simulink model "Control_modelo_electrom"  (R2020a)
settings: Solver=VariableStepAuto  StartTime=0.0  StopTime=10.0  RelTol=1e-3
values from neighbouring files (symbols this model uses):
  b = 0.1    [Comando_linmod.m]
  k = 0.8    [Comando_linmod.m]
  kf = 0.45    [Comando_linmod.m]
  kv = 0.45    [Comando_linmod.m]
  L = 0.1    [Comando_linmod.m]
  m = 0.15    [Comando_linmod.m]
  M = 5    [Comando_linmod.m]
  R = 0.25    [Comando_linmod.m]
undefined symbols (not defined in the file or in its folder): den, num
libraries: simulink x2

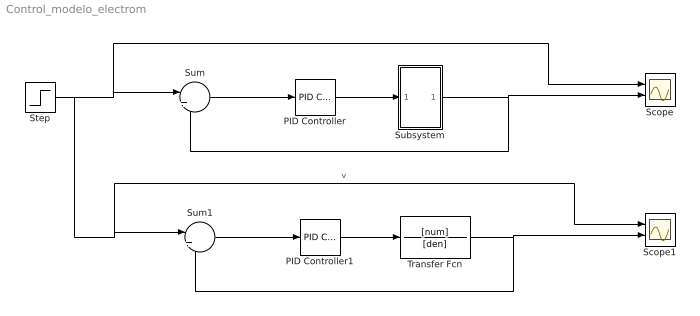
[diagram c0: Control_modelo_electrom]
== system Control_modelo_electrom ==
  PID Controller : simulink/Continuous/PID Controller  Controller=PID  Form=Parallel  TimeDomain=Continuous-time  UseExternalTs=off  SampleTime=-1  IntegratorMethod=Forward Euler  FilterMethod=Forward Euler  ControllerParametersSource=internal  P=1  I=1  D=0  UseFilter=on  N=100  TunerSelectOption=Transfer Function Based (PID Tuner App)  InitialConditionSource=internal  InitialConditionForIntegrator=0  InitialConditionForFilter=0  DifferentiatorICPrevScaledInput=0  ExternalReset=none  TrackingMode=off  Kt=1  LimitOutput=off  UpperSaturationLimit=inf  LowerSaturationLimit=-inf  LinearizeAsGain=on  AntiWindupMode=none  Kb=1  POutMin=[]  POutMax=[]  IOutMin=[]  IOutMax=[]  DOutMin=[]  DOutMax=[]  NOutMin=[]  NOutMax=[]  SumOutMin=[]  SumOutMax=[]  SaturationOutMin=[]  SaturationOutMax=[]  PParamMin=[]  PParamMax=[]  IParamMin=[]  IParamMax=[]  DParamMin=[]  DParamMax=[]  NParamMin=[]  NParamMax=[]  KbParamMin=[]  KbParamMax=[]  KtParamMin=[]  KtParamMax=[]  KbOutMin=[]  KbOutMax=[]  KtOutMin=[]  KtOutMax=[]  IntegratorOutMin=[]  IntegratorOutMax=[]  FilterOutMin=[]  FilterOutMax=[]  SumI1OutMin=[]  SumI1OutMax=[]  SumI2OutMin=[]  SumI2OutMax=[]  SumI3OutMin=[]  SumI3OutMax=[]  SumI4OutMin=[]  SumI4OutMax=[]  SumDOutMin=[]  SumDOutMax=[]  DifferentiatorOutMin=[]  DifferentiatorOutMax=[]  FilterDiffOutCoefMin=[]  FilterDiffOutCoefMax=[]  ReciprocalOutMin=[]  ReciprocalOutMax=[]  SumDenOutMin=[]  SumDenOutMax=[]  SumNumOutMin=[]  SumNumOutMax=[]  DivideOutMin=[]  DivideOutMax=[]  UdiffTsProdOutMin=[]  UdiffTsProdOutMax=[]  NTsProdOutMin=[]  NTsProdOutMax=[]  UintegralTsProdOutMin=[]  UintegralTsProdOutMax=[]  UngainTsProdOutMin=[]  UngainTsProdOutMax=[]  IntegratorContinuousStateAttributes=''  IntegratorStateMustResolveToSignalObject=off  IntegratorRTWStateStorageClass=Auto  FilterContinuousStateAttributes=''  FilterStateMustResolveToSignalObject=off  FilterRTWStateStorageClass=Auto  ParallelPVariant=InternalParameters  IdealPVariant=Disabled  IVariant=InternalParameters  DVariant=InternalParameters  IntegratorVariant=Continuous  SatVariant=Disabled  AWVariant=Passthrough  PCopyVariant=Disabled  TRVariant=Disabled  FdbkBlocksVariant=Forward  IdealPFdbkVariant=Disabled  SatFdbkVariant=Disabled  DerivativeFilterVariant=ContFilter  NVariant=InternalParameters  NCopyVariant=Disabled  FilterICVariant=InternalICsFilter  IntegratorICVariant=InternalICs  ExternalResetVariant=Disabled  TRSumVariant=Passthrough  SumFdbkVariant=Disabled  SumVariant=Sum_PID  TsampFilterVariant=InternalTs  TsampNgainVariant=Passthrough  TsampIntegralVariant=Passthrough
  PID Controller1 : simulink/Continuous/PID Controller  Controller=PID  Form=Parallel  TimeDomain=Continuous-time  UseExternalTs=off  SampleTime=-1  IntegratorMethod=Forward Euler  FilterMethod=Forward Euler  ControllerParametersSource=internal  P=1  I=1  D=0  UseFilter=on  N=100  TunerSelectOption=Transfer Function Based (PID Tuner App)  InitialConditionSource=internal  InitialConditionForIntegrator=0  InitialConditionForFilter=0  DifferentiatorICPrevScaledInput=0  ExternalReset=none  TrackingMode=off  Kt=1  LimitOutput=off  UpperSaturationLimit=inf  LowerSaturationLimit=-inf  LinearizeAsGain=on  AntiWindupMode=none  Kb=1  POutMin=[]  POutMax=[]  IOutMin=[]  IOutMax=[]  DOutMin=[]  DOutMax=[]  NOutMin=[]  NOutMax=[]  SumOutMin=[]  SumOutMax=[]  SaturationOutMin=[]  SaturationOutMax=[]  PParamMin=[]  PParamMax=[]  IParamMin=[]  IParamMax=[]  DParamMin=[]  DParamMax=[]  NParamMin=[]  NParamMax=[]  KbParamMin=[]  KbParamMax=[]  KtParamMin=[]  KtParamMax=[]  KbOutMin=[]  KbOutMax=[]  KtOutMin=[]  KtOutMax=[]  IntegratorOutMin=[]  IntegratorOutMax=[]  FilterOutMin=[]  FilterOutMax=[]  SumI1OutMin=[]  SumI1OutMax=[]  SumI2OutMin=[]  SumI2OutMax=[]  SumI3OutMin=[]  SumI3OutMax=[]  SumI4OutMin=[]  SumI4OutMax=[]  SumDOutMin=[]  SumDOutMax=[]  DifferentiatorOutMin=[]  DifferentiatorOutMax=[]  FilterDiffOutCoefMin=[]  FilterDiffOutCoefMax=[]  ReciprocalOutMin=[]  ReciprocalOutMax=[]  SumDenOutMin=[]  SumDenOutMax=[]  SumNumOutMin=[]  SumNumOutMax=[]  DivideOutMin=[]  DivideOutMax=[]  UdiffTsProdOutMin=[]  UdiffTsProdOutMax=[]  NTsProdOutMin=[]  NTsProdOutMax=[]  UintegralTsProdOutMin=[]  UintegralTsProdOutMax=[]  UngainTsProdOutMin=[]  UngainTsProdOutMax=[]  IntegratorContinuousStateAttributes=''  IntegratorStateMustResolveToSignalObject=off  IntegratorRTWStateStorageClass=Auto  FilterContinuousStateAttributes=''  FilterStateMustResolveToSignalObject=off  FilterRTWStateStorageClass=Auto  ParallelPVariant=InternalParameters  IdealPVariant=Disabled  IVariant=InternalParameters  DVariant=InternalParameters  IntegratorVariant=Continuous  SatVariant=Disabled  AWVariant=Passthrough  PCopyVariant=Disabled  TRVariant=Disabled  FdbkBlocksVariant=Forward  IdealPFdbkVariant=Disabled  SatFdbkVariant=Disabled  DerivativeFilterVariant=ContFilter  NVariant=InternalParameters  NCopyVariant=Disabled  FilterICVariant=InternalICsFilter  IntegratorICVariant=InternalICs  ExternalResetVariant=Disabled  TRSumVariant=Passthrough  SumFdbkVariant=Disabled  SumVariant=Sum_PID  TsampFilterVariant=InternalTs  TsampNgainVariant=Passthrough  TsampIntegralVariant=Passthrough
  Scope : Scope  NumInputPorts=2
  Scope1 : Scope  NumInputPorts=2
  Step : Step  SampleTime=0
  Subsystem : Subsystem
  Sum : Sum  Inputs=|+-
  Sum1 : Sum  Inputs=|+-
  Transfer Fcn : TransferFcn  Numerator=[num]  Denominator=[den]
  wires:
  Subsystem/1(dx/dt) -> Sum/2, Scope/2
  PID Controller/1 -> Subsystem/1(v)
  Sum/1 -> PID Controller/1
  Sum1/1 -> PID Controller1/1
  PID Controller1/1 -> Transfer Fcn/1
  Step/1 -> Scope1/1, Sum1/1, Sum/1, Scope/1  "v"
  Transfer Fcn/1 -> Scope1/2, Sum1/2

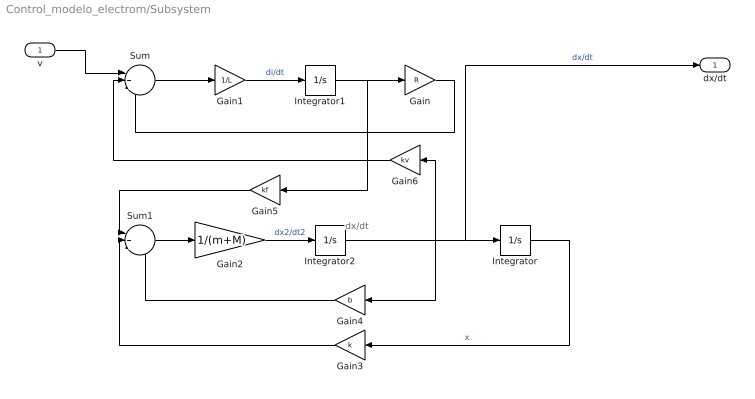
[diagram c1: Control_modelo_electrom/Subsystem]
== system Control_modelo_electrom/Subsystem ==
  note: dx/dt
  v : Inport
  Gain : Gain  Gain=R
  Gain1 : Gain  Gain=1/L
  Gain2 : Gain  Gain=1/(m+M)
  Gain3 : Gain  Gain=k
  Gain4 : Gain  Gain=b
  Gain5 : Gain  Gain=kf
  Gain6 : Gain  Gain=kv
  Integrator : Integrator
  Integrator1 : Integrator
  Integrator2 : Integrator
  Sum : Sum  Inputs=|+--
  Sum1 : Sum  Inputs=|+--
  dx/dt : Outport
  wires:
  Integrator2/1 -> Gain4/1, Gain6/1, dx/dt/1, Integrator/1  "dx/dt"
  Gain2/1 -> Integrator2/1  "dx2/dt2"
  Integrator/1 -> Gain3/1  "x"
  Gain3/1 -> Sum1/2
  Integrator1/1 -> Gain5/1, Gain/1  "i"
  Gain4/1 -> Sum1/3
  Gain/1 -> Sum/3
  Sum1/1 -> Gain2/1
  Gain1/1 -> Integrator1/1  "di/dt"
  Gain5/1 -> Sum1/1
  Gain6/1 -> Sum/2
  Sum/1 -> Gain1/1
  v/1 -> Sum/1
